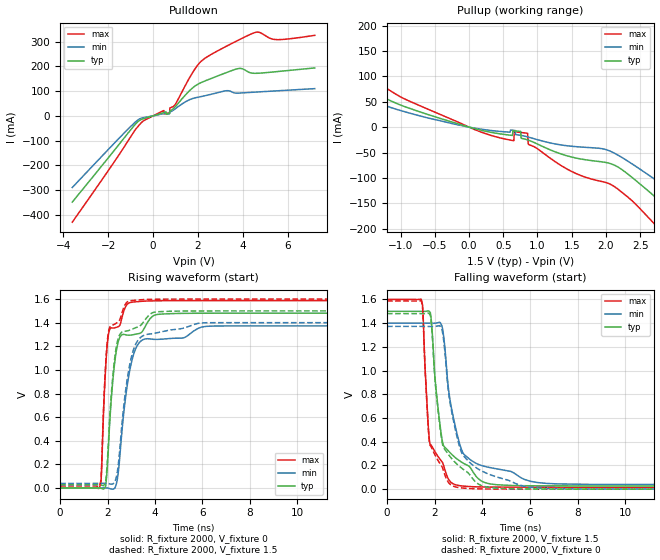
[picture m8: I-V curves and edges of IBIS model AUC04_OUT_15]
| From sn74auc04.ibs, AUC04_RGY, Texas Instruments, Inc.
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[Model]   AUC04_OUT_15
Model_type  Output
Vref =   0
Rref =   2000
Cref =   15p
Vmeas =   0.75
| variable   typ   min   max
C_comp   3.5pF   NA   NA
| C_pullup   7.01pF   2.00pF   19.70pF
| C_pulldown   7.08pF   4.51pF   15.46pF
[Temperature Range]   40   100   -40
| Ambient temperature   25   85   -40
[Voltage range]   1.5   1.4   1.6
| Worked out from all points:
|   slope of the pulldown table from 0 to 0.225 V, typ, clamps not added: 37.3 ohm
|   slope of the pullup table from 0 to 0.225 V, typ, clamps not added: 29.6 ohm
|   rising waveform, R_fixture 2000, V_fixture 0: 20-80 % time 366ps typ, 529ps min, 241ps max; typ from 0 V to 1.48 V
|   falling waveform, R_fixture 2000, V_fixture 1.5: 20-80 % time 644ps typ, 719ps min, 417ps max; typ from 1.5 V to 0.027 V
|   rising waveform, R_fixture 2000, V_fixture 1.5: 20-80 % time 361ps typ, 522ps min, 237ps max; typ from 0.027 V to 1.5 V
|   falling waveform, R_fixture 2000, V_fixture 0: 20-80 % time 630ps typ, 782ps min, 397ps max; typ from 1.48 V to 0 V
[Pulldown]
| AUC04_OUT_15
|   Voltage   I(typ)   I(min)   I(max)
-3.6V     -348.4mA   -289.5mA   -429.6mA
-665mV    -22.33mA   -15.81mA   -42.01mA
480mV     13.54mA    9.64mA     21.5mA
735mV     9.284mA    14.92mA    12.28mA
750mV     20.66mA    15.42mA    31.62mA
980mV     36.38mA    28.08mA    45.45mA
1.775V    114mA      70.34mA    177.1mA
2.235V    138.2mA    79.83mA    227.7mA
3.81V     191.5mA    91.9mA     306.5mA
4.58V     172mA      96.1mA     337.9mA
5.485V    178.5mA    101mA      308.2mA
7.2V      193.7mA    110mA      325.3mA
[Pullup]
| AUC04_OUT_15
|   Voltage   I(typ)   I(min)   I(max)
-3.6V     266mA      208.2mA    314.3mA
-2.885V   197.2mA    157.7mA    242.1mA
-2.5V     161mA      126.6mA    203.2mA
-900mV    38.43mA    28.74mA    52.85mA
390mV     -11.89mA   -7.641mA   -18.98mA
855mV     -25.04mA   -19.21mA   -12.06mA
870mV     -25.74mA   -19.76mA   -33.77mA
1.35V     -53.08mA   -35.2mA    -76.07mA
2.125V    -74.89mA   -51.34mA   -117.2mA
2.825V    -149.3mA   -113mA     -207mA
3.65V     -245.1mA   -192.4mA   -322.4mA
7.2V      -652.9mA   -541.5mA   -802.5mA
[Ramp]
| AUC04_OUT_15
| variable   typ   min   max
dV/dt_r   0.89/3.69E-10   0.83/5.31E-10   0.96/2.44E-10
dV/dt_f   0.89/6.42E-10   0.82/7.25E-10   0.95/4.17E-10
R_load = 2000
[Rising Waveform]
| AUC04_OUT_15
R_fixture =   2000
C_fixture =   0
L_fixture =   0
V_fixture =   0
V_fixture_min = 0
V_fixture_max = 0
|   Time   V(typ)   V(min)   V(max)
0s        9.392nV    35.9nV     957pV
1.675ns   -253.8uV   682.7uV    13.81mV
1.735ns   -2.484mV   802uV      96.32mV
1.915ns   13.07mV    1.018mV    1.003V
2.035ns   338.1mV    -1.569mV   1.296V
2.395ns   1.191V     55.61mV    1.362V
2.935ns   1.294V     995.8mV    1.569V
3.465ns   1.325V     1.253V     1.581V
6.145ns   1.48V      1.369V     1.587V
22.2ns    1.481V     1.373V     1.587V
[Falling Waveform]
| AUC04_OUT_15
R_fixture =   2000
C_fixture =   0
L_fixture =   0
V_fixture =   1.5
V_fixture_min = 1.4
V_fixture_max = 1.6
|   Time   V(typ)   V(min)   V(max)
0s        1.5V       1.4V       1.6V
1.43ns    1.5V       1.4V       1.603V
1.495ns   1.5V       1.4V       1.535V
1.605ns   1.5V       1.4V       989.2mV
1.79ns    1.495V     1.399V     395.2mV
2.31ns    418.2mV    1.372V     230.2mV
2.855ns   267.9mV    537.7mV    38.23mV
3.55ns    164.6mV    240.7mV    21.26mV
6.32ns    28.36mV    55.62mV    16.65mV
22.2ns    27.24mV    38.79mV    16.43mV
[Rising Waveform]
| AUC04_OUT_15
R_fixture =   2000
C_fixture =   0
L_fixture =   0
V_fixture =   1.5
V_fixture_min = 1.4
V_fixture_max = 1.6
|   Time   V(typ)   V(min)   V(max)
0s        27.17mV    38.75mV    16.4mV
1.67ns    27.05mV    39.36mV    29.33mV
1.73ns    25.16mV    39.47mV    97.2mV
1.915ns   49.66mV    39.63mV    1.029V
2.03ns    363.7mV    37.48mV    1.31V
2.37ns    1.195V     92.65mV    1.396V
2.87ns    1.333V     973.5mV    1.581V
3.425ns   1.383V     1.28V      1.594V
5.89ns    1.499V     1.397V     1.6V
22.2ns    1.5V       1.4V       1.6V
[Falling Waveform]
| AUC04_OUT_15
R_fixture =   2000
C_fixture =   0
L_fixture =   0
V_fixture =   0
V_fixture_min = 0
V_fixture_max = 0
|   Time   V(typ)   V(min)   V(max)
0s        1.481V     1.373V     1.587V
1.43ns    1.48V      1.373V     1.59V
1.495ns   1.48V      1.373V     1.52V
1.605ns   1.48V      1.372V     979.9mV
1.79ns    1.474V     1.372V     380.9mV
2.3ns     408mV      1.349V     192.8mV
2.805ns   236.8mV    559.8mV    22.99mV
3.555ns   97.86mV    209.5mV    4.53mV
5.935ns   1.481mV    17.71mV    299.8uV
22.2ns    70.88uV    36.46uV    29.59uV
